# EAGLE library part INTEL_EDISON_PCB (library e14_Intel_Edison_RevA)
Intel Edison Compute Module. Ideal for creating your own PCB to host an Edison. Created for www.element14.com by Dave of Young Circuit Designs. Note: 70-pin connector on the Edison is a 1.5mm-tall Hirose plug DF40C-70DP-0.4V(51) Mating Hirose receptacle connectors of varying heights include the following Hirose part numbers: 1.5mm-tall: DF40C-70DS-0.4V(51) 2.0mm-tall: DF40C(2.0)-70DS-0.4V(51) 3.0mm-tall: DF40CG(3.0)-70DS-0.4V(51) The host board will sit flush with the Edison's shield if the 1.5mm-tall receptacle is used. More information can be found on the Intel Edison Compute Module Hardware Guide.
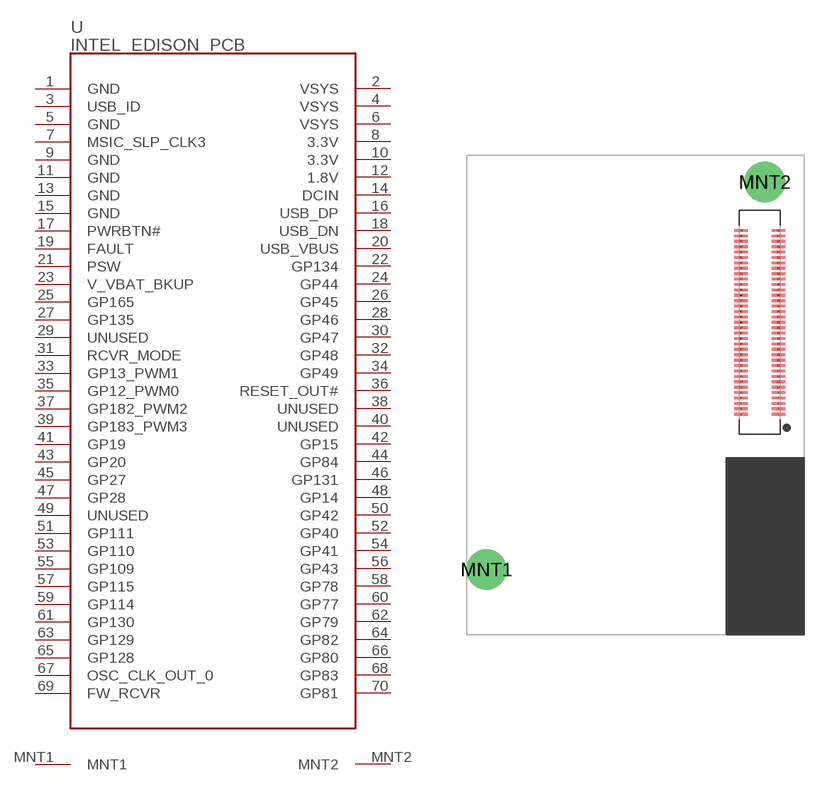
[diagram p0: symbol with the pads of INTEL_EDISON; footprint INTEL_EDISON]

Designator prefix -

## INTEL_EDISON_PCB  [INTEL_EDISON]
1  GND
2  VSYS
3  USB_ID
4  VSYS
5  GND
6  VSYS
7  MSIC_SLP_CLK3
8  3.3V
9  GND
10  3.3V
11  GND
12  1.8V
13  GND
14  DCIN
15  GND
16  USB_DP
17  PWRBTN#
18  USB_DN
19  FAULT
20  USB_VBUS
21  PSW
22  GP134
23  V_VBAT_BKUP
24  GP44
25  GP165
26  GP45
27  GP135
28  GP46
29  UNUSED
30  GP47
31  RCVR_MODE
32  GP48
33  GP13_PWM1
34  GP49
35  GP12_PWM0
36  RESET_OUT#
37  GP182_PWM2
38  UNUSED
39  GP183_PWM3
40  UNUSED
41  GP19
42  GP15
43  GP20
44  GP84
45  GP27
46  GP131
47  GP28
48  GP14
49  UNUSED
50  GP42
51  GP111
52  GP40
53  GP110
54  GP41
55  GP109
56  GP43
57  GP115
58  GP78
59  GP114
60  GP77
61  GP130
62  GP79
63  GP129
64  GP82
65  GP128
66  GP80
67  OSC_CLK_OUT_0
68  GP83
69  FW_RCVR
70  GP81
MNT1  MNT1
MNT2  MNT2

## Footprint INTEL_EDISON (pad centres in mm)
Intel Edison Compute Module. Ideal for creating your own PCB to host an Edison. Created for www.element14.com by Dave of Young Circuit Designs. Note: 70-pin connector on the Edison is a 1.5mm-tall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
smd 1 x 0.2: 1 21.62,11.5; 2 18.84,11.5; 3 21.62,11.9; 4 18.84,11.9; 5 21.62,12.3; 6 18.84,12.3; 7 21.62,12.7; 8 18.84,12.7; 9 21.62,13.1; 10 18.84,13.1; 11 21.62,13.5; 12 18.84,13.5; 13 21.62,13.9; 14 18.84,13.9; 15 21.62,14.3; 16 18.84,14.3; 17 21.62,14.7; 18 18.84,14.7; 19 21.62,15.1; 20 18.84,15.1; 21 21.62,15.5; 22 18.84,15.5; 23 21.62,15.9; 24 18.84,15.9; 25 21.62,16.3; 26 18.84,16.3; 27 21.62,16.7; 28 18.84,16.7; 29 21.62,17.1; 30 18.84,17.1; 31 21.62,17.5; 32 18.84,17.5; 33 21.62,17.9; 34 18.84,17.9; 35 21.62,18.3; 36 18.84,18.3; 37 21.62,18.7; 38 18.84,18.7; 39 21.62,19.1; 40 18.84,19.1; 41 21.62,19.5; 42 18.84,19.5; 43 21.62,19.9; 44 18.84,19.9; 45 21.62,20.3; 46 18.84,20.3; 47 21.62,20.7; 48 18.84,20.7; 49 21.62,21.1; 50 18.84,21.1; 51 21.62,21.5; 52 18.84,21.5; 53 21.62,21.9; 54 18.84,21.9; 55 21.62,22.3; 56 18.84,22.3; 57 21.62,22.7; 58 18.84,22.7; 59 21.62,23.1; 60 18.84,23.1; 61 21.62,23.5; 62 18.84,23.5; 63 21.62,23.9; 64 18.84,23.9; 65 21.62,24.3; 66 18.84,24.3; 67 21.62,24.7; 68 18.84,24.7; 69 21.62,25.1; 70 18.84,25.1
drill 2: MNT1 0,0; MNT2 20.6,28.69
